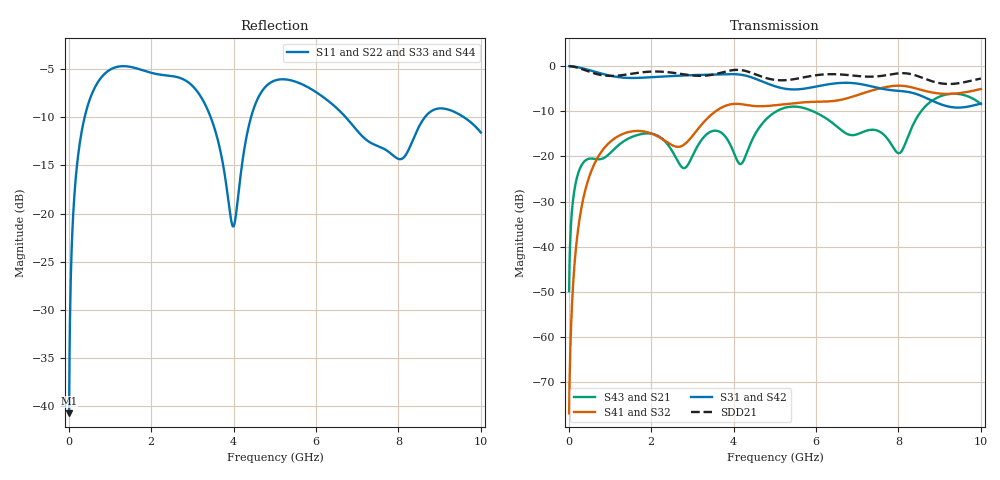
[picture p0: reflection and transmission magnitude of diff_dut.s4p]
# HZ S RI R 50
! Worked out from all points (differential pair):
!   1000 points, 10 MHz to 10 GHz, reference 50 ohm
!   strongest paths, dB at 10 MHz, 2.51 GHz, 5.01 GHz, 7.51 GHz, 10 GHz:
!     S31: 0.0, -2.2, -4.5, -4.8, -8.3
!     S42: 0.0, -2.2, -4.5, -4.8, -8.3
!     S41: -76.9, -17.5, -8.7, -5.0, -5.1
!     S32: -76.9, -17.5, -8.7, -5.0, -5.1
!     S43: -49.8, -18.8, -10.2, -14.3, -8.4
!     S21: -49.8, -18.8, -10.2, -14.3, -8.4
!   taken as a pair (ports 1,2 in; 3,4 out), SDD21 dB: 0.0, -1.4, -3.0, -2.2, -2.7
!   lowest |S11| = -40.7 dB at 10 MHz (marker M1), VSWR 1.02, Z = 50 - j0.917 ohm
!   |S11| at or under -10 dB: 3.445 GHz to 4.424 GHz (979.2 MHz wide, 24.9 % of centre); 6.72 GHz to 8.641 GHz (1.921 GHz wide, 25 % of centre); 9.586 GHz to end of sweep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
1e7  -0.000413 -0.00918  0.000156 0.00321  0.9991 -0.0268  6.43e-05 -0.000128
     0.000156 0.00321  -0.000413 -0.00918  6.43e-05 -0.000128  0.9991 -0.0268
     0.9991 -0.0268  6.43e-05 -0.000128  -0.000413 -0.00918  0.000156 0.00321
     6.43e-05 -0.000128  0.9991 -0.0268  0.000156 0.00321  -0.000413 -0.00918
3.1e8  -0.1925 -0.1794  0.0553 0.0575  0.6525 -0.6942  0.00281 -0.027
       0.0553 0.0575  -0.1925 -0.1794  0.00281 -0.027  0.6525 -0.6942
       0.6525 -0.6942  0.00281 -0.027  -0.1925 -0.1794  0.0553 0.0575
       0.00281 -0.027  0.6525 -0.6942  0.0553 0.0575  -0.1925 -0.1794
1.1e9  -0.2663 0.5045  0.1103 0.0472  -0.6804 -0.3587  -0.0771 0.1366
       0.1103 0.0472  -0.2663 0.5045  -0.0771 0.1366  -0.6804 -0.3587
       -0.6804 -0.3587  -0.0771 0.1366  -0.2663 0.5045  0.1103 0.0472
       -0.0771 0.1366  -0.6804 -0.3587  0.1103 0.0472  -0.2663 0.5045
2.71e9  0.00875 -0.5045  -0.0699 -0.038  0.785 0.0216  -0.0236 -0.1268
        -0.0699 -0.038  0.00875 -0.5045  -0.0236 -0.1268  0.785 0.0216
        0.785 0.0216  -0.0236 -0.1268  0.00875 -0.5045  -0.0699 -0.038
        -0.0236 -0.1268  0.785 0.0216  -0.0699 -0.038  0.00875 -0.5045
3.99e9  -0.0841 -0.0162  0.0123 -0.1141  -0.814 -0.0515  -0.0195 0.3809
        0.0123 -0.1141  -0.0841 -0.0162  -0.0195 0.3809  -0.814 -0.0515
        -0.814 -0.0515  -0.0195 0.3809  -0.0841 -0.0162  0.0123 -0.1141
        -0.0195 0.3809  -0.814 -0.0515  0.0123 -0.1141  -0.0841 -0.0162
5.26e9  -0.075 0.4909  0.3408 0.069  0.5506 0.1092  0.0477 -0.3767
        0.3408 0.069  -0.075 0.4909  0.0477 -0.3767  0.5506 0.1092
        0.5506 0.1092  0.0477 -0.3767  -0.075 0.4909  0.3408 0.069
        0.0477 -0.3767  0.5506 0.1092  0.3408 0.069  -0.075 0.4909
1e10  0.2613 -0.0314  0.0868 -0.3723  -0.055 0.3812  0.5582 -0.0133
      0.0868 -0.3723  0.2613 -0.0314  0.5582 -0.0133  -0.055 0.3812
      -0.055 0.3812  0.5582 -0.0133  0.2613 -0.0314  0.0868 -0.3723
      0.5582 -0.0133  -0.055 0.3812  0.0868 -0.3723  0.2613 -0.0314
